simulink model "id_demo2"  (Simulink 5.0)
settings: Solver=ode45  SolverMode=SingleTasking  StartTime=0.0  StopTime=10  RelTol=1e-3  AbsTol=1e-3
libraries: simulink x1

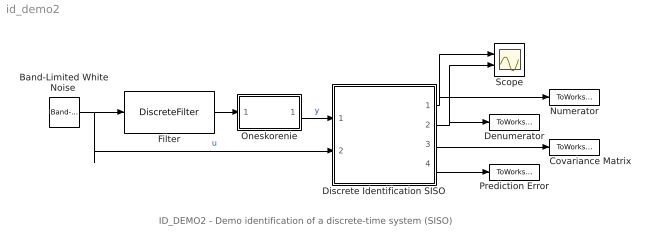
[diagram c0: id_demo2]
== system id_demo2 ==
  note: ID_DEMO2 - Demo identification of a discrete-time system (SISO)
  "Band-Limited White Noise " : simulink/Sources/Band-Limited White Noise  Cov=[0.1]  Ts=0.1  seed=[23341]
  Covariance Matrix : ToWorkspace  VariableName=CovMatrix  SaveFormat=Array
  Denumerator : ToWorkspace  VariableName=A  SaveFormat=Array
  Discrete Identification SISO : Subsystem  mask(Discrete Identification){par1=[2,2], Ds=[0], par2=[0.985,0.01], poc=[0 0 0 0], kov=[10e6], ts=[1]}
      mask prompts: par1 "Degrees of numerator and denominator -  [dn, dd]:"; Ds "Discrete time delay - [D]:"; par2 "Exponential forgetting and Bittanti's correction - [L, d]:"; poc "Initial parameter estimates - [theta(1) ... theta(n)]:"; kov "Covariance matrix (see help, standard - [10e6]):"; ts "Sampling time - [ts]:"
      mask help: Discrete identification Authors: Lubos Cirka and Miroslav Fikar 1998 - 2006
      mask init:
      | % State-space realisation of discete-time MIMO filters
      | %
      | % Input:
      | %    y1(k), ..., yn(k), u1(k), ..., um(k)
      | % Output:
      | %    y(k), y(k-1), y(k-2) ..., u(k-1-Ds), ...
      | 
      | % State-space realisation of the output filter
      | 
      | cit=par1(1);men=par1(2);L=par2(1);d=par2(2);n=cit+men;m=1;in=1;out=1;
      | A0=zeros(men*out);
      | A0(out+1:men*out,1:(men-1)*out)=eye((men-1)*out);
      | Ay=A0;
      | 
      | B0=-eye(out);
      | B1=zeros((men-1)*out,out);
      | By=[B0;B1];
      | 
      | C0=zeros(out,men*out);
      | C1=eye(men*out);
      | Cy=[C0;C1];
      | 
      | D1=eye(out);
      | D2=zeros(men*out,out);
      | Dy=[D1;D2];
      | 
      | % State-space realisation of the input filter
      | 
      | a0=zeros(in,(cit+Ds)*in);
      | a1=eye((cit+Ds-1)*in);
      | a2=zeros((cit+Ds-1)*in,in);
      | Au=[a0;[a1 a2]];
      | 
      | b0=eye(in);
      | b1=zeros((cit+Ds-1)*in,in);
      | Bu=[b0;b1];
      | 
      | c0=zeros(cit*in,Ds*in);
      | c1=eye(cit*in);
      | Cu=[c0 c1];
      | 
      | Du=zeros(cit*in,in);
  Filter : DiscreteFilter  Numerator=[0 0.8 0.2]  Denominator=[1 -0.5 0.06]
  Numerator : ToWorkspace  VariableName=B  SaveFormat=Array
  Oneskorenie : Subsystem  mask(Time Delay){LDd=[0], LDts=[1]}
      mask prompts: LDd "Discrete time delay - [D]:"; LDts "Sampling time - [ts]:"
      mask help: Discrete time delay Authors: Lubos Cirka and Miroslav Fikar 1998 - 2004
      mask init:
      | A=[zeros(1,1+LDd);eye(LDd),zeros(LDd,1)];B=[1;zeros(LDd,1)]; if LDd==0; C=0; D=1; else C=[zeros(1,LDd-1) 1 0]; D=0; end;
  Prediction Error : ToWorkspace  VariableName=PredError  SaveFormat=Array
  Scope : Scope  NumInputPorts=2
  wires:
  Oneskorenie/1(u(k-d)) -> Discrete Identification SISO/1(y)  "y"
  "Band-Limited White Noise "/1 -> Filter/1, Discrete Identification SISO/2(u)  "u"
  Filter/1 -> Oneskorenie/1(u(k))
  Discrete Identification SISO/4(prediction error) -> Prediction Error/1
  Discrete Identification SISO/3("Covariance matrix ") -> Covariance Matrix/1
  Discrete Identification SISO/2(A) -> Denumerator/1, Scope/2
  Discrete Identification SISO/1(B) -> Numerator/1, Scope/1

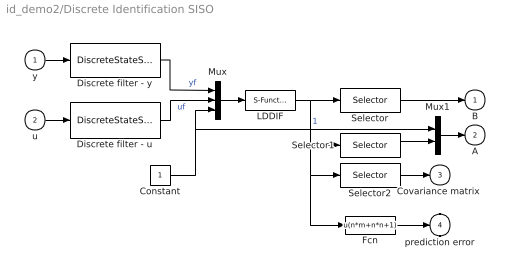
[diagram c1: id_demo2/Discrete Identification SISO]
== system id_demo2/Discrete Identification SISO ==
  y : Inport
  u : Inport  Port=2
  Constant : Constant
  Discrete filter - u : DiscreteStateSpace  A=Au  B=Bu  C=Cu  D=Du  SampleTime=ts
  Discrete filter - y : DiscreteStateSpace  A=Ay  B=By  C=Cy  D=Dy  SampleTime=ts
  Fcn : Fcn  Expr=u(n*m+n*n+1)
  LDDIF : S-Function  FunctionName=lddif_s  Parameters=m ,n+1 ,L ,d, [poc 0], kov, ts
  Mux : Mux  Inputs=3
  Mux1 : Mux  Inputs=2
  Selector : Selector  Elements=[men+1:1:men+cit]  InputPortWidth=(n+1)*m+(n+1)*(n+1)+m
  Selector1 : Selector  Elements=[1:1:men]  InputPortWidth=(n+1)*m+(n+1)*(n+1)+m
  Selector2 : Selector  Elements=[(n+1)*m+1:1:(n+1)*m+(n+1)*(n+1)]  InputPortWidth=(n+1)*m+(n+1)*(n+1)+m
  B : Outport  InitialOutput=0
  A : Outport  Port=2  InitialOutput=0
  "Covariance matrix " : Outport  Port=3  InitialOutput=0
  prediction error : Outport  Port=4  InitialOutput=0
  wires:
  Constant/1 -> Mux1/1, Mux/3  "1"
  Selector1/1 -> Mux1/2
  Fcn/1 -> prediction error/1
  Selector2/1 -> "Covariance matrix "/1
  Mux1/1 -> A/1
  Mux/1 -> LDDIF/1
  Selector/1 -> B/1
  y/1 -> Discrete filter - y/1
  u/1 -> Discrete filter - u/1
  Discrete filter - y/1 -> Mux/1  "yf"
  Discrete filter - u/1 -> Mux/2  "uf"
  LDDIF/1 -> Selector/1, Selector1/1, Selector2/1, Fcn/1

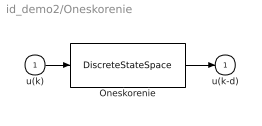
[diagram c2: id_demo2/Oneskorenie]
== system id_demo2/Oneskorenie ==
  u(k) : Inport
  Oneskorenie : DiscreteStateSpace  A=A  B=B  C=C  D=D  SampleTime=LDts
  u(k-d) : Outport  InitialOutput=0
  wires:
  Oneskorenie/1 -> u(k-d)/1
  u(k)/1 -> Oneskorenie/1
